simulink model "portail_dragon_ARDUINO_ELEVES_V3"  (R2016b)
settings: Solver=FixedStepAuto  StartTime=0.0  StopTime=inf  FixedStep=1e-3  RelTol=1e-3  EnableMultiTasking=on
libraries: arduinolib x11, simulink x3

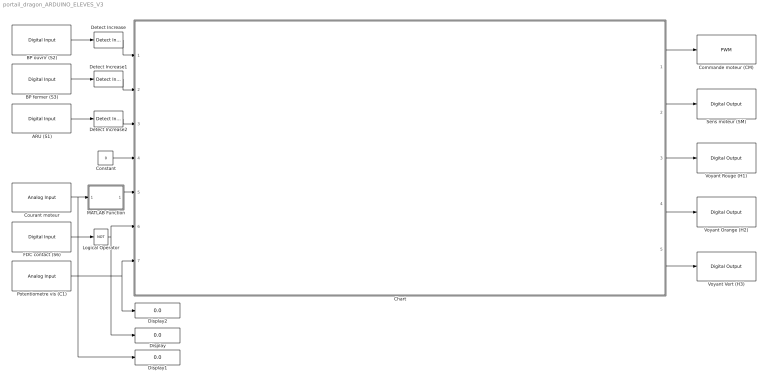
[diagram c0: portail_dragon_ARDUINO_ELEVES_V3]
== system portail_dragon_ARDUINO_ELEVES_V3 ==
  ARU (S1) : arduinolib/Digital Input  pinNumber=40  sampleTime=0.01  blockPlatform=arduino
  BP fermer (S3) : arduinolib/Digital Input  pinNumber=44  sampleTime=0.01  blockPlatform=arduino
  BP ouvrir (S2) : arduinolib/Digital Input  pinNumber=42  sampleTime=0.01  blockPlatform=arduino
  Chart : Stateflow chart  TreatAsAtomicUnit=on
  Commande moteur (CM) : arduinolib/PWM  pinNumber=8  blockPlatform=arduino
  Constant : Constant  Value=0
  Courant moteur : arduinolib/Analog Input  pinNumber=2  sampleTime=0.01  blockPlatform=arduino
  Detect Increase : simulink/Logic and Bit Operations/Detect Increase  vinit=0.0  OutDataTypeStr=boolean
  Detect Increase1 : simulink/Logic and Bit Operations/Detect Increase  vinit=0.0  OutDataTypeStr=boolean
  Detect Increase2 : simulink/Logic and Bit Operations/Detect Increase  vinit=0.0  OutDataTypeStr=boolean
  Display : Display
  Display1 : Display
  Display2 : Display
  FDC contact (S6) : arduinolib/Digital Input  pinNumber=50  sampleTime=0.01  blockPlatform=arduino
  Logical Operator : Logic  Operator=NOT  AllPortsSameDT=off  OutDataTypeStr=boolean
  MATLAB Function : MATLAB Function  TreatAsAtomicUnit=on
  Potentiometre vis (C1) : arduinolib/Analog Input  pinNumber=1  sampleTime=0.01  blockPlatform=arduino
  Sens moteur (SM) : arduinolib/Digital Output  pinNumber=26  blockPlatform=arduino
  Voyant Orange (H2) : arduinolib/Digital Output  pinNumber=30  blockPlatform=arduino
  Voyant Rouge (H1) : arduinolib/Digital Output  pinNumber=32  blockPlatform=arduino
  Voyant Vert (H3) : arduinolib/Digital Output  pinNumber=28  blockPlatform=arduino
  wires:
  Detect Increase/1 -> Chart/1(bp_ouvrir)
  Detect Increase1/1 -> Chart/2(bp_fermer)
  Constant/1 -> Chart/4(br_auto)
  MATLAB Function/1(courant_max) -> Chart/5(courant_max)
  BP ouvrir (S2)/1 -> Detect Increase/1
  BP fermer (S3)/1 -> Detect Increase1/1
  Courant moteur/1 -> MATLAB Function/1(courant), Display1/1
  FDC contact (S6)/1 -> Logical Operator/1
  Potentiometre vis (C1)/1 -> Chart/7(pos_vis), Display2/1
  Chart/1(v_mot) -> Commande moteur (CM)/1
  Chart/3(H1) -> Voyant Rouge (H1)/1
  Chart/4(H2) -> Voyant Orange (H2)/1
  Chart/5(H3) -> Voyant Vert (H3)/1
  ARU (S1)/1 -> Detect Increase2/1
  Detect Increase2/1 -> Chart/3(ARU)
  Chart/2(s_mot) -> Sens moteur (SM)/1
  Logical Operator/1 -> Chart/6(fdc_ferme), Display/1

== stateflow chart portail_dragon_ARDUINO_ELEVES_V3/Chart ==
  data: v_mot output; s_mot output; H1 output; H2 output; H3 output; bp_ouvrir input; bp_fermer input; ARU input; br_auto input; courant_max input; fdc_ferme input; pos_vis input

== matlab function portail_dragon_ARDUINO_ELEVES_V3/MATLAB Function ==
function courant_max = fcn(courant)

if courant > 620
    courant_max = 1;
else
    courant_max =0;
end
